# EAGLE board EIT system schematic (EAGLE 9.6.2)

Size 100 x 80 mm. Coordinates in mm from the lower left corner, seen from the top.
Outline: 0,0 100,0 100,80 0,80 0,0
Copper layers (1*16): Top 0.035mm / dielectric 1.5mm / Bottom 0.035mm
Design rules "default": minimum track width 6mil, minimum drill 0.35mm, track to track 6mil, track to pad 6mil, pad to pad 6mil, via to via 6mil, smd to smd 6mil, copper to edge 40mil, drill to drill 6mil, minimum pad ring 10mil, minimum via ring 8mil, stop-mask expansion 4mil, vias tented up to drill 0mil, thermal gap 10mil

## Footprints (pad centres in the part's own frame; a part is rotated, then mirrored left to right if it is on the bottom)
1X02 = drill 1.016 long: 1 -1.27,0; 2 1.27,0
C0805 = smd 1.3 x 1.5: 1 -0.95,0; 2 0.95,0
1X05 = drill 1.016 long: 1 -5.08,0; 2 -2.54,0; 3 0,0; 4 2.54,0; 5 5.08,0
SO14 = smd 0.66 x 2.032: 1 -3.81,-3.073; 2 -2.54,-3.073; 3 -1.27,-3.073; 4 0,-3.073; 5 1.27,-3.073; 6 2.54,-3.073; 7 3.81,-3.073; 8 3.81,3.073; 9 2.54,3.073; 10 1.27,3.073; 11 0,3.073; 12 -1.27,3.073; 13 -2.54,3.073; 14 -3.81,3.073
1X01 = drill 1.016 octagon: 1 0,0
2X16 = drill 1.016 octagon: 1 -19.05,-1.27; 2 -19.05,1.27; 3 -16.51,-1.27; 4 -16.51,1.27; 5 -13.97,-1.27; 6 -13.97,1.27; 7 -11.43,-1.27; 8 -11.43,1.27; 9 -8.89,-1.27; 10 -8.89,1.27; 11 -6.35,-1.27; 12 -6.35,1.27; 13 -3.81,-1.27; 14 -3.81,1.27; 15 -1.27,-1.27; 16 -1.27,1.27; 17 1.27,-1.27; 18 1.27,1.27; 19 3.81,-1.27; 20 3.81,1.27; 21 6.35,-1.27; 22 6.35,1.27; 23 8.89,-1.27; 24 8.89,1.27; 25 11.43,-1.27; 26 11.43,1.27; 27 13.97,-1.27; 28 13.97,1.27; 29 16.51,-1.27; 30 16.51,1.27; 31 19.05,-1.27; 32 19.05,1.27
2X08 = drill 1.016 octagon: 1 -8.89,-1.27; 2 -8.89,1.27; 3 -6.35,-1.27; 4 -6.35,1.27; 5 -3.81,-1.27; 6 -3.81,1.27; 7 -1.27,-1.27; 8 -1.27,1.27; 9 1.27,-1.27; 10 1.27,1.27; 11 3.81,-1.27; 12 3.81,1.27; 13 6.35,-1.27; 14 6.35,1.27; 15 8.89,-1.27; 16 8.89,1.27
1_05X2MM = drill 1.016 pad 1.3 square: 1 -4,0 | drill 1.016 pad 1.3: 2 -2,0; 3 0,0; 4 2,0; 5 4,0
M0805 = smd 1.3 x 1.6: 1 -0.95,0; 2 0.95,0
SOIC127P599X175-8N = smd 1.97 x 0.6: 1 -2.47,1.905; 2 -2.47,0.635; 3 -2.47,-0.635; 4 -2.47,-1.905; 5 2.47,-1.905; 6 2.47,-0.635; 7 2.47,0.635; 8 2.47,1.905
DIP254P762X533-8 = drill 1.118 square: 1 -7.62,7.62 | drill 1.118: 2 -7.62,5.08; 3 -7.62,2.54; 4 -7.62,0; 5 0,0; 6 0,2.54; 7 0,5.08; 8 0,7.62
SOIC127P1030X265-24N = smd 2.06 x 0.6: 1 -4.64,6.985; 2 -4.64,5.715; 3 -4.64,4.445; 4 -4.64,3.175; 5 -4.64,1.905; 6 -4.64,0.635; 7 -4.64,-0.635; 8 -4.64,-1.905; 9 -4.64,-3.175; 10 -4.64,-4.445; 11 -4.64,-5.715; 12 -4.64,-6.985; 13 4.64,-6.985; 14 4.64,-5.715; 15 4.64,-4.445; 16 4.64,-3.175; 17 4.64,-1.905; 18 4.64,-0.635; 19 4.64,0.635; 20 4.64,1.905; 21 4.64,3.175; 22 4.64,4.445; 23 4.64,5.715; 24 4.64,6.985
DIP1016W50P254L742H480Q6 = drill 0.82 square: 1 -5.08,2.54 | drill 0.82: 2 -5.08,0; 3 -5.08,-2.54; 4 5.08,-2.54; 5 5.08,0; 6 5.08,2.54

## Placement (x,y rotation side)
ADC1-2  [1X02]  not placed on the board
C3  1uf  [C0805]  not placed on the board
C4  1uf  [C0805]  not placed on the board
DEMUX3  [1X05]  not placed on the board
DEMUX4  [1X05]  not placed on the board
IC2  7404D  [SO14]  not placed on the board
JP2  [1X01]  74.93,12.7 0 top
JP3  [2X16]  not placed on the board
JP6  [2X08]  not placed on the board
MUX1_2  [1_05X2MM]  not placed on the board
R1  10K  [M0805]  not placed on the board
R2  10k  [M0805]  not placed on the board
R3  10k  [M0805]  not placed on the board
R4  10K  [M0805]  not placed on the board
R5  [M0805]  not placed on the board
R6  10k  [M0805]  not placed on the board
R7  10k  [M0805]  not placed on the board
R8  [M0805]  not placed on the board
R9  [M0805]  not placed on the board
R10  [M0805]  not placed on the board
R11  10K  [M0805]  not placed on the board
R12  10k  [M0805]  not placed on the board
R13  10k  [M0805]  not placed on the board
R14  10K  [M0805]  not placed on the board
R15  [M0805]  not placed on the board
R16  10k  [M0805]  not placed on the board
R17  10k  [M0805]  not placed on the board
R18  10K  [M0805]  not placed on the board
R19  10k  [M0805]  not placed on the board
R20  10k  [M0805]  not placed on the board
R21  [M0805]  not placed on the board
R22  [M0805]  not placed on the board
R23  [M0805]  not placed on the board
R24  [M0805]  not placed on the board
R25  [M0805]  not placed on the board
R26  [M0805]  not placed on the board
R27  [M0805]  not placed on the board
R28  10K  [M0805]  not placed on the board
R29  [M0805]  not placed on the board
R30  10k  [M0805]  not placed on the board
R31  10k  [M0805]  not placed on the board
R32  10K  [M0805]  not placed on the board
R33  10k  [M0805]  not placed on the board
R34  10k  [M0805]  not placed on the board
R35  10K  [M0805]  not placed on the board
R36  [M0805]  not placed on the board
R37  10k  [M0805]  not placed on the board
R38  10k  [M0805]  not placed on the board
R39  10K  [M0805]  not placed on the board
R40  10k  [M0805]  not placed on the board
R41  10k  [M0805]  not placed on the board
R42  10K  [M0805]  not placed on the board
R43  [M0805]  not placed on the board
R44  10k  [M0805]  not placed on the board
R45  10k  [M0805]  not placed on the board
R46  10K  [M0805]  not placed on the board
R47  10k  [M0805]  not placed on the board
R48  10k  [M0805]  not placed on the board
R49  10K  [M0805]  not placed on the board
R50  [M0805]  not placed on the board
R51  10k  [M0805]  not placed on the board
R52  10k  [M0805]  not placed on the board
R53  10K  [M0805]  not placed on the board
R54  10k  [M0805]  not placed on the board
R55  10k  [M0805]  not placed on the board
R56  10K  [M0805]  not placed on the board
R57  [M0805]  not placed on the board
R58  10k  [M0805]  not placed on the board
R59  10k  [M0805]  not placed on the board
R60  10K  [M0805]  not placed on the board
R61  10k  [M0805]  not placed on the board
R62  10k  [M0805]  not placed on the board
R63  10K  [M0805]  not placed on the board
R64  [M0805]  not placed on the board
R65  10k  [M0805]  not placed on the board
R66  10k  [M0805]  not placed on the board
R67  10K  [M0805]  not placed on the board
R68  10k  [M0805]  not placed on the board
R69  10k  [M0805]  not placed on the board
R70  10K  [M0805]  not placed on the board
R71  [M0805]  not placed on the board
R72  10k  [M0805]  not placed on the board
R73  10k  [M0805]  not placed on the board
R74  10K  [M0805]  not placed on the board
R75  10k  [M0805]  not placed on the board
R76  10k  [M0805]  not placed on the board
R77  10K  [M0805]  not placed on the board
R78  [M0805]  not placed on the board
R79  10k  [M0805]  not placed on the board
R80  10k  [M0805]  not placed on the board
R81  10K  [M0805]  not placed on the board
R82  10k  [M0805]  not placed on the board
R83  10k  [M0805]  not placed on the board
R84  10K  [M0805]  not placed on the board
R85  [M0805]  not placed on the board
R86  10k  [M0805]  not placed on the board
R87  10k  [M0805]  not placed on the board
R88  10K  [M0805]  not placed on the board
R89  10k  [M0805]  not placed on the board
R90  10k  [M0805]  not placed on the board
R91  10K  [M0805]  not placed on the board
R92  [M0805]  not placed on the board
R93  10k  [M0805]  not placed on the board
R94  10k  [M0805]  not placed on the board
R95  10K  [M0805]  not placed on the board
R96  10k  [M0805]  not placed on the board
R97  10k  [M0805]  not placed on the board
R98  10K  [M0805]  not placed on the board
R99  [M0805]  not placed on the board
R100  10k  [M0805]  not placed on the board
R101  10k  [M0805]  not placed on the board
R102  10K  [M0805]  not placed on the board
R103  10k  [M0805]  not placed on the board
R104  10k  [M0805]  not placed on the board
R105  10K  [M0805]  not placed on the board
R106  [M0805]  not placed on the board
R107  10k  [M0805]  not placed on the board
R108  10k  [M0805]  not placed on the board
R109  10K  [M0805]  not placed on the board
R110  10k  [M0805]  not placed on the board
R111  10k  [M0805]  not placed on the board
R112  10K  [M0805]  not placed on the board
R113  [M0805]  not placed on the board
R114  10k  [M0805]  not placed on the board
R115  10k  [M0805]  82.55,29.21 0 top
R116  10K  [M0805]  not placed on the board
R117  10k  [M0805]  not placed on the board
R118  10k  [M0805]  not placed on the board
R119  10K  [M0805]  not placed on the board
R120  [M0805]  not placed on the board
R121  10k  [M0805]  not placed on the board
R122  10k  [M0805]  not placed on the board
SUPPLY  [1X02]  not placed on the board
U1  OPA657U  [SOIC127P599X175-8N]  93.98,72.39 0 top
U2  OPA657U  [SOIC127P599X175-8N]  88.9,17.78 0 top
U3  AD781JNZ  [DIP254P762X533-8]  not placed on the board
U4  AD781JNZ  [DIP254P762X533-8]  not placed on the board
U5  OPA657U  [SOIC127P599X175-8N]  45.72,17.78 0 top
U6  OPA657U  [SOIC127P599X175-8N]  44.45,52.07 0 top
U7  OPA657U  [SOIC127P599X175-8N]  not placed on the board
U8  OPA657U  [SOIC127P599X175-8N]  not placed on the board
U9  CD74HCT4067M  [SOIC127P1030X265-24N]  24.13,27.94 0 top
U10  CD74HCT4067M  [SOIC127P1030X265-24N]  not placed on the board
U11  AD781JNZ  [DIP254P762X533-8]  not placed on the board
U12  AD781JNZ  [DIP254P762X533-8]  not placed on the board
U13  AD781JNZ  [DIP254P762X533-8]  not placed on the board
U14  AD781JNZ  [DIP254P762X533-8]  not placed on the board
U15  AD781JNZ  [DIP254P762X533-8]  not placed on the board
U16  AD781JNZ  [DIP254P762X533-8]  not placed on the board
U17  AD781JNZ  [DIP254P762X533-8]  not placed on the board
U18  AD781JNZ  [DIP254P762X533-8]  not placed on the board
U19  AD781JNZ  [DIP254P762X533-8]  not placed on the board
U20  AD781JNZ  [DIP254P762X533-8]  not placed on the board
U21  OPA657U  [SOIC127P599X175-8N]  not placed on the board
U22  AD781JNZ  [DIP254P762X533-8]  not placed on the board
U23  OPA657U  [SOIC127P599X175-8N]  not placed on the board
U24  H11AA4M  [DIP1016W50P254L742H480Q6]  not placed on the board
U25  H11AA4M  [DIP1016W50P254L742H480Q6]  not placed on the board
U26  CD74HCT4067M  [SOIC127P1030X265-24N]  not placed on the board
U27  CD74HCT4067M  [SOIC127P1030X265-24N]  not placed on the board
U28  OPA657U  [SOIC127P599X175-8N]  not placed on the board
U29  OPA657U  [SOIC127P599X175-8N]  not placed on the board
U30  OPA657U  [SOIC127P599X175-8N]  not placed on the board
U31  OPA657U  [SOIC127P599X175-8N]  not placed on the board
U32  OPA657U  [SOIC127P599X175-8N]  not placed on the board
U33  OPA657U  [SOIC127P599X175-8N]  not placed on the board
U34  OPA657U  [SOIC127P599X175-8N]  not placed on the board
U35  OPA657U  [SOIC127P599X175-8N]  60.96,12.7 0 top
U36  OPA657U  [SOIC127P599X175-8N]  17.78,67.31 0 top
U37  OPA657U  [SOIC127P599X175-8N]  44.45,69.85 0 top
U38  OPA657U  [SOIC127P599X175-8N]  not placed on the board
U39  OPA657U  [SOIC127P599X175-8N]  not placed on the board
U40  AD781JNZ  [DIP254P762X533-8]  not placed on the board
U41  AD781JNZ  [DIP254P762X533-8]  not placed on the board
U42  AD781JNZ  [DIP254P762X533-8]  not placed on the board
U43  AD781JNZ  [DIP254P762X533-8]  not placed on the board
U44  AD781JNZ  [DIP254P762X533-8]  not placed on the board
U45  AD781JNZ  [DIP254P762X533-8]  not placed on the board
U46  AD781JNZ  [DIP254P762X533-8]  not placed on the board
U47  AD781JNZ  [DIP254P762X533-8]  not placed on the board
U48  AD781JNZ  [DIP254P762X533-8]  not placed on the board
U49  AD781JNZ  [DIP254P762X533-8]  not placed on the board
U50  AD781JNZ  [DIP254P762X533-8]  not placed on the board
U51  AD781JNZ  [DIP254P762X533-8]  not placed on the board
U52  AD781JNZ  [DIP254P762X533-8]  not placed on the board
U53  AD781JNZ  [DIP254P762X533-8]  not placed on the board
U54  AD781JNZ  [DIP254P762X533-8]  not placed on the board
U55  AD781JNZ  [DIP254P762X533-8]  not placed on the board
U56  AD781JNZ  [DIP254P762X533-8]  not placed on the board
U57  AD781JNZ  [DIP254P762X533-8]  not placed on the board
U58  AD781JNZ  [DIP254P762X533-8]  not placed on the board
U59  OPA657U  [SOIC127P599X175-8N]  not placed on the board
U60  OPA657U  [SOIC127P599X175-8N]  not placed on the board
U61  OPA657U  [SOIC127P599X175-8N]  not placed on the board
U62  OPA657U  [SOIC127P599X175-8N]  not placed on the board
U63  OPA657U  [SOIC127P599X175-8N]  not placed on the board
U64  OPA657U  [SOIC127P599X175-8N]  not placed on the board
U65  OPA657U  [SOIC127P599X175-8N]  not placed on the board
U66  OPA657U  [SOIC127P599X175-8N]  not placed on the board
U67  OPA657U  [SOIC127P599X175-8N]  not placed on the board
U68  OPA657U  [SOIC127P599X175-8N]  91.44,60.96 0 top
U69  OPA657U  [SOIC127P599X175-8N]  83.82,72.39 0 top
U70  OPA657U  [SOIC127P599X175-8N]  57.15,71.12 0 top
U71  OPA657U  [SOIC127P599X175-8N]  not placed on the board
U72  OPA657U  [SOIC127P599X175-8N]  not placed on the board
U73  OPA657U  [SOIC127P599X175-8N]  not placed on the board
U74  OPA657U  [SOIC127P599X175-8N]  not placed on the board
U75  OPA657U  [SOIC127P599X175-8N]  not placed on the board
U76  OPA657U  [SOIC127P599X175-8N]  not placed on the board
U77  OPA657U  [SOIC127P599X175-8N]  not placed on the board
U78  OPA657U  [SOIC127P599X175-8N]  not placed on the board
U79  OPA657U  [SOIC127P599X175-8N]  not placed on the board
U80  OPA657U  [SOIC127P599X175-8N]  not placed on the board
U81  OPA657U  [SOIC127P599X175-8N]  not placed on the board
U82  OPA657U  [SOIC127P599X175-8N]  not placed on the board
U83  OPA657U  [SOIC127P599X175-8N]  71.12,71.12 0 top
U84  OPA657U  [SOIC127P599X175-8N]  31.75,68.58 0 top
U85  OPA657U  [SOIC127P599X175-8N]  81.28,48.26 0 top
U86  OPA657U  [SOIC127P599X175-8N]  not placed on the board
U87  OPA657U  [SOIC127P599X175-8N]  not placed on the board
U88  OPA657U  [SOIC127P599X175-8N]  not placed on the board

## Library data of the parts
ADC1-2 DEMUX3 DEMUX4 JP2 JP3 JP6 MUX1_2 SUPPLY = pinhead
C3 C4 = rcl; SPICEPREFIX: C
IC2 = 74xx-eu
R1-R122 = rcl; SPICEPREFIX: R
U1 U2 U5-U8 U21 U23 U28-U39 U59-U88 = OPA657U; DESCRIPTION: 1.6GHz, Low Noise, FET-Input Operational Amplifier 8-SOIC -40 to 85; DIGI-KEY_PART_NUMBER: OPA657UB-ND; MF: Texas Instruments; MP: OPA657U; PACKAGE: SOIC-8 Texas Instruments; PURCHASE-URL: https://pricing.snapeda.com/search/part/OPA657U/?ref=eda
U3 U4 U11-U20 U22 U40-U58 = AD781JNZ; AVAILABILITY: Good; DESCRIPTION: Sample and Hold Amplifier 1 Circuit 8-PDIP; MF: Analog Devices; MP: AD781JNZ; PACKAGE: PDIP-8 Analog Devices; PRICE: None; PURCHASE-URL: https://pricing.snapeda.com/search/part/AD781JNZ/?ref=eda
U9 U10 U26 U27 = CD74HCT4067M; AVAILABILITY: Good; DESCRIPTION: 5-V, 16:1, 1-channel analog multiplexer with TTL inputs 24-SOIC -55 to 125; MF: Texas Instruments; MP: CD74HCT4067M; PACKAGE: SOIC-24 Texas Instruments; PRICE: None; PURCHASE-URL: https://pricing.snapeda.com/search/part/CD74HCT4067M/?ref=eda
U24 U25 = H11AA4M; AVAILABILITY: Good; DESCRIPTION: AC-IN 1-CH Transistor With Base DC-OUT 6-Pin PDIP Bag; MF: ON Semiconductor; MP: H11AA4M; PACKAGE: PDIP-6 ON Semiconductor; PRICE: None; PURCHASE-URL: https://pricing.snapeda.com/search/part/H11AA4M/?ref=eda

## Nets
0: C3.1 C4.1 R7.1 R17.1 R22.2 R23.2 R31.1 R38.1 R45.1 R52.1 R59.1 R66.1 R73.1 R80.1 R87.1 R94.1 R101.1 R108.1 R115.1 R122.1 U3.3 U4.3 U9.12 U10.12 U11.3 U12.3 U13.3 U14.3 U15.3 U16.3 U17.3 U18.3 U19.3 U20.3 U22.3 U24.2 U25.2 U26.12 U27.12 U40.3 U41.3 U42.3 U43.3 U44.3 U45.3 U46.3 U47.3 U48.3 U49.3 U50.3 U51.3 U52.3 U53.3 U54.3 U55.3 U56.3 U57.3 U58.3
+5V: U27.24
+12V: C4.2 SUPPLY.1 U13.1 U14.1 U17.1 U20.1 U40.1 U41.1 U42.1 U44.1 U45.1 U46.1 U47.1 U48.1 U53.1 U54.1 U55.1 U56.1
-5V: U21.4
-12V: C3.2 SUPPLY.2 U13.5 U14.5 U17.5 U20.5 U40.5 U41.5 U42.5 U44.5 U45.5 U46.5 U47.5 U48.5 U49.1 U53.5 U54.5 U55.5 U56.5
D3E: DEMUX3.1
D3S0: DEMUX3.2 U9.10
D3S1: DEMUX3.3 U9.11
D3S2: DEMUX3.4 U9.14
D3S3: DEMUX3.5 U9.13
D4E: DEMUX4.1
D4S0: DEMUX4.2
D4S1: DEMUX4.3
D4S2: DEMUX4.4
D4S3: DEMUX4.5
E: MUX1_2.1 U26.15
GND: IC2.7
I0: JP3.2 U48.8
I1: JP3.4 U10.8 U45.8
I2: JP3.6 U10.7 U53.8
I3: JP3.8 U10.6 U44.8
I4: JP3.10 U10.5 U46.8
I5: JP3.12 U10.4 U12.8
I6: JP3.14 U4.8 U10.3
I7: JP3.16 U3.8 U10.2
I8: JP3.18 U10.23 U22.8
I9: JP3.20 U10.22 U18.8
I10: JP3.22 U10.21 U57.8
I11: JP3.24 U10.20 U50.8
I12: JP3.26 U10.19 U51.8
I13: JP3.28 U10.18 U43.8
I14: JP3.30 U10.17 U58.8
I15: JP3.32 U10.16 U52.8
IO: U10.9
M1I0: U26.9 U48.2
M1I1: U26.8 U45.2
M1I2: U26.7 U53.2
M1I3: U26.6 U44.2
M1I4: U26.5 U46.2
M1I5: U12.2 U26.4
M1I6: U4.2 U26.3
M1I7: U3.2 U26.2
M1I8: U22.2 U26.23
M1I9: U18.2 U26.22
M1I10: U26.21 U57.2
M1I11: U26.20 U50.2
M1I12: U26.19 U51.2
M1I13: U26.18 U43.2
M1I14: U26.17 U58.2
M1I15: U26.16 U52.2
M2I0: U11.2 U27.9
M2I1: U15.2 U27.8
M2I2: U14.2 U27.7
M2I3: U13.2 U27.6
M2I4: U27.5 U54.2
M2I5: U27.4 U40.2
M2I6: U27.3 U47.2
M2I7: U27.2 U55.2
M2I8: U19.2 U27.23
M2I9: U16.2 U27.22
M2I10: U17.2 U27.21
M2I11: U20.2 U27.20
M2I12: U27.19 U56.2
M2I13: U27.18 U49.2
M2I14: U27.17 U42.2
M2I15: U27.16 U41.2
N$1: U9.24
N$3: U1.4
N$4: U1.7
N$5: U2.4
N$6: U2.7
N$7: U5.4
N$8: U5.7
N$9: U23.4
N$10: U23.7
N$11: U25.4 U27.1
N$12: ADC1-2.2 U10.1
N$14: IC2.1 JP2.1
N$15: U41.7
N$16: U52.1
N$17: JP3.1 U11.8
N$18: R2.1 R3.2 U2.2
N$19: JP3.3 U15.8
N$20: R1.1 R2.2 U1.2
N$21: JP3.5 U14.8
N$22: R3.1 R5.2 U2.6
N$23: JP3.7 U13.8
N$24: R5.1 R7.2 U5.3
N$25: U40.7
N$26: JP3.17 U19.8
N$27: JP3.19 U16.8
N$28: R1.2 R4.2 U1.6
N$29: R4.1 R6.2 U5.2
N$30: U4.7
N$31: U49.5
N$32: U4.1
N$33: JP3.21 U17.8
N$34: R6.1 U5.6 U9.22
N$35: JP3.23 U20.8
N$36: JP3.25 U56.8
N$37: JP3.27 U49.8
N$39: U4.5
N$40: U3.1
N$41: U3.7
N$43: U53.7
N$45: U44.7
N$47: U46.7
N$49: U12.1
N$50: U12.7
N$51: U12.5
N$54: U3.5
N$55: U11.1
N$56: U11.7
N$57: U42.7
N$58: U11.5
N$59: U15.1
N$60: U15.7
N$61: U52.7
N$62: U15.5
N$63: U14.7
N$64: U52.5
N$65: U49.7
N$66: U56.7
N$67: U54.7
N$68: U13.7
N$69: U58.1
N$70: U55.7
N$71: U47.7
N$72: U20.7
N$73: JP3.9 U54.8
N$74: JP3.11 U40.8
N$75: JP3.13 U47.8
N$76: JP3.15 U55.8
N$77: U58.7
N$78: U17.7
N$79: U6.4
N$80: U16.1
N$81: U16.7
N$82: U58.5
N$83: U16.5
N$84: U19.1
N$85: U19.7
N$86: U43.1
N$87: U19.5
N$88: JP3.29 U42.8
N$89: JP3.31 U41.8
N$90: U43.7
N$91: U6.7
N$92: U43.5
N$93: U51.1
N$94: U51.7
N$95: U7.4
N$96: U51.5
N$97: U50.1
N$98: U50.7
N$99: U7.7
N$100: U50.5
N$101: U57.1
N$102: U57.7
N$103: U8.4
N$104: U57.5
N$105: U18.1
N$106: U18.7
N$107: U8.7
N$108: U18.5
N$109: U22.1
N$110: U22.7
N$111: R37.1 U9.7 U33.6
N$112: U22.5
N$121: R8.2 R10.1 U21.3
N$122: R21.2 R22.1 U21.2
N$123: R9.2 R21.1 U21.6
N$124: R8.1 R9.1 U24.1
N$125: R23.1 R26.2 U23.3
N$126: R24.1 R27.2 U23.2
N$127: R25.2 R27.1 U23.6
N$128: R25.1 R26.1 U25.1
N$129: R24.2
N$130: U25.5
N$131: U24.4 U26.1
N$132: U80.4
N$133: U27.10
N$134: U27.11
N$135: U27.15
N$136: U27.14
N$137: U27.13
N$138: R93.1 U9.8 U76.6
N$139: R12.1 R13.2 U7.2
N$140: R11.1 R12.2 U6.2
N$141: R13.1 R15.2 U7.6
N$142: R15.1 R17.2 U8.3
N$143: R11.2 R14.2 U6.6
N$144: R14.1 R16.2 U8.2
N$145: R16.1 U8.6 U9.18
N$146: U28.4
N$147: U28.7
N$148: U29.4
N$149: U29.7
N$150: U30.4
N$151: U30.7
N$152: R86.1 U9.9 U73.6
N$153: U10.24
N$154: R19.1 R20.2 U29.2
N$155: R18.1 R19.2 U28.2
N$156: R20.1 R29.2 U29.6
N$157: R29.1 R31.2 U30.3
N$158: R18.2 R28.2 U28.6
N$159: R28.1 R30.2 U30.2
N$160: R30.1 U9.3 U30.6
N$161: U31.4
N$162: U31.7
N$163: U32.4
N$164: U32.7
N$165: U33.4
N$166: U33.7
N$167: U10.10
N$168: U10.11
N$169: R33.1 R34.2 U32.2
N$170: R32.1 R33.2 U31.2
N$171: R34.1 R36.2 U32.6
N$172: R36.1 R38.2 U33.3
N$173: R32.2 R35.2 U31.6
N$174: R35.1 R37.2 U33.2
N$175: U10.13
N$176: U34.4
N$177: U34.7
N$178: U35.4
N$179: U35.7
N$180: U36.4
N$181: U36.7
N$182: U10.14
N$184: R40.1 R41.2 U35.2
N$185: R39.1 R40.2 U34.2
N$186: R41.1 R43.2 U35.6
N$187: R43.1 R45.2 U36.3
N$188: R39.2 R42.2 U34.6
N$189: R42.1 R44.2 U36.2
N$190: R44.1 U9.21 U36.6
N$191: U37.4
N$192: U37.7
N$193: U38.4
N$194: U38.7
N$195: U39.4
N$196: U39.7
N$199: R47.1 R48.2 U38.2
N$200: R46.1 R47.2 U37.2
N$201: R48.1 R50.2 U38.6
N$202: R50.1 R52.2 U39.3
N$203: R46.2 R49.2 U37.6
N$204: R49.1 R51.2 U39.2
N$205: R51.1 U9.20 U39.6
N$206: U59.4
N$207: U59.7
N$208: U60.4
N$209: U60.7
N$210: U61.4
N$211: U61.7
N$214: R54.1 R55.2 U60.2
N$215: R53.1 R54.2 U59.2
N$216: R55.1 R57.2 U60.6
N$217: R57.1 R59.2 U61.3
N$218: R53.2 R56.2 U59.6
N$219: R56.1 R58.2 U61.2
N$220: R58.1 U9.16 U61.6
N$221: U62.4
N$222: U62.7
N$223: U63.4
N$224: U63.7
N$225: U64.4
N$226: U64.7
N$229: R61.1 R62.2 U63.2
N$230: R60.1 R61.2 U62.2
N$231: R62.1 R64.2 U63.6
N$232: R64.1 R66.2 U64.3
N$233: R60.2 R63.2 U62.6
N$234: R63.1 R65.2 U64.2
N$235: R65.1 U9.17 U64.6
N$236: U65.4
N$237: U65.7
N$238: U66.4
N$239: U66.7
N$240: U67.4
N$241: U67.7
N$244: R68.1 R69.2 U66.2
N$245: R67.1 R68.2 U65.2
N$246: R69.1 R71.2 U66.6
N$247: R71.1 R73.2 U67.3
N$248: R67.2 R70.2 U65.6
N$249: R70.1 R72.2 U67.2
N$250: R72.1 U9.4 U67.6
N$251: U68.4
N$252: U68.7
N$253: U69.4
N$254: U69.7
N$255: U70.4
N$256: U70.7
N$259: R75.1 R76.2 U69.2
N$260: R74.1 R75.2 U68.2
N$261: R76.1 R78.2 U69.6
N$262: R78.1 R80.2 U70.3
N$263: R74.2 R77.2 U68.6
N$264: R77.1 R79.2 U70.2
N$265: R79.1 U9.5 U70.6
N$266: U71.4
N$267: U71.7
N$268: U72.4
N$269: U72.7
N$270: U73.4
N$271: U73.7
N$274: R82.1 R83.2 U72.2
N$275: R81.1 R82.2 U71.2
N$276: R83.1 R85.2 U72.6
N$277: R85.1 R87.2 U73.3
N$278: R81.2 R84.2 U71.6
N$279: R84.1 R86.2 U73.2
N$281: U74.4
N$282: U74.7
N$283: U75.4
N$284: U75.7
N$285: U76.4
N$286: U76.7
N$289: R89.1 R90.2 U75.2
N$290: R88.1 R89.2 U74.2
N$291: R90.1 R92.2 U75.6
N$292: R92.1 R94.2 U76.3
N$293: R88.2 R91.2 U74.6
N$294: R91.1 R93.2 U76.2
N$296: U77.4
N$297: U77.7
N$298: U21.7
N$299: U78.4
N$300: U78.7
N$301: U79.4
N$302: U79.7
N$305: R96.1 R97.2 U78.2
N$306: R95.1 R96.2 U77.2
N$307: R97.1 R99.2 U78.6
N$308: R99.1 R101.2 U79.3
N$309: R95.2 R98.2 U77.6
N$310: R98.1 R100.2 U79.2
N$311: R100.1 U9.23 U79.6
N$312: U80.7
N$313: U81.4
N$314: U81.7
N$315: U82.4
N$316: U82.7
N$319: R103.1 R104.2 U81.2
N$320: R102.1 R103.2 U80.2
N$321: R104.1 R106.2 U81.6
N$322: R106.1 R108.2 U82.3
N$323: R102.2 R105.2 U80.6
N$324: R105.1 R107.2 U82.2
N$325: R107.1 U9.19 U82.6
N$326: U83.4
N$327: U83.7
N$328: U84.4
N$329: U84.7
N$330: U85.4
N$331: U85.7
N$334: R110.1 R111.2 U84.2
N$335: R109.1 R110.2 U83.2
N$336: R111.1 R113.2 U84.6
N$337: R113.1 R115.2 U85.3
N$338: R109.2 R112.2 U83.6
N$339: R112.1 R114.2 U85.2
N$340: R114.1 U9.2 U85.6
N$341: U86.4
N$342: U86.7
N$343: U87.4
N$344: U87.7
N$345: U88.4
N$346: U88.7
N$349: R117.1 R118.2 U87.2
N$350: R116.1 R117.2 U86.2
N$351: R118.1 R120.2 U87.6
N$352: R120.1 R122.2 U88.3
N$353: R116.2 R119.2 U86.6
N$354: R119.1 R121.2 U88.2
N$355: R121.1 U9.6 U88.6
N$361: ADC1-2.1 U9.1
N$367: U9.15
S0: MUX1_2.2 U26.10
S1: MUX1_2.3 U26.11
S2: MUX1_2.4 U26.14
S3: MUX1_2.5 U26.13
STATUS: IC2.2 U45.7 U48.7
V1: JP6.1 U72.3 U77.3
V2: JP6.2 U78.3 U80.3
V3: JP6.3 U81.3 U83.3
V4: JP6.4 U84.3 U86.3
V5: JP6.5 U1.3 U87.3
V6: JP6.6 U2.3 U6.3
V7: JP6.7 U7.3 U28.3
V8: JP6.8 U29.3 U31.3
V9: JP6.9 U32.3 U34.3
V10: JP6.10 U35.3 U62.3
V11: JP6.11 U63.3 U65.3
V12: JP6.12 U66.3 U74.3
V13: JP6.13 U37.3 U75.3
V14: JP6.14 U38.3 U59.3
V15: JP6.15 U60.3 U68.3
V16: JP6.16 U69.3 U71.3
VCC: IC2.14 U26.24
VSOURCE: R10.2 U24.5

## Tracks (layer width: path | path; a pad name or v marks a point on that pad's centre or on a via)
0  (57 unrouted)
+12V  (17 unrouted)
-12V  (18 unrouted)
D3S0  (1 unrouted)
D3S1  (1 unrouted)
D3S2  (1 unrouted)
D3S3  (1 unrouted)
E  (1 unrouted)
I0  (1 unrouted)
I1  (2 unrouted)
I2  (2 unrouted)
I3  (2 unrouted)
I4  (2 unrouted)
I5  (2 unrouted)
I6  (2 unrouted)
I7  (2 unrouted)
I8  (2 unrouted)
I9  (2 unrouted)
I10  (2 unrouted)
I11  (2 unrouted)
I12  (2 unrouted)
I13  (2 unrouted)
I14  (2 unrouted)
I15  (2 unrouted)
M1I0  (1 unrouted)
M1I1  (1 unrouted)
M1I2  (1 unrouted)
M1I3  (1 unrouted)
M1I4  (1 unrouted)
M1I5  (1 unrouted)
M1I6  (1 unrouted)
M1I7  (1 unrouted)
M1I8  (1 unrouted)
M1I9  (1 unrouted)
M1I10  (1 unrouted)
M1I11  (1 unrouted)
M1I12  (1 unrouted)
M1I13  (1 unrouted)
M1I14  (1 unrouted)
M1I15  (1 unrouted)
M2I0  (1 unrouted)
M2I1  (1 unrouted)
M2I2  (1 unrouted)
M2I3  (1 unrouted)
M2I4  (1 unrouted)
M2I5  (1 unrouted)
M2I6  (1 unrouted)
M2I7  (1 unrouted)
M2I8  (1 unrouted)
M2I9  (1 unrouted)
M2I10  (1 unrouted)
M2I11  (1 unrouted)
M2I12  (1 unrouted)
M2I13  (1 unrouted)
M2I14  (1 unrouted)
M2I15  (1 unrouted)
N$11  (1 unrouted)
N$12  (1 unrouted)
N$14  (1 unrouted)
N$17  (1 unrouted)
N$18  (2 unrouted)
N$19  (1 unrouted)
N$20  (2 unrouted)
N$21  (1 unrouted)
N$22  (2 unrouted)
N$23  (1 unrouted)
N$24  (2 unrouted)
N$26  (1 unrouted)
N$27  (1 unrouted)
N$28  (2 unrouted)
N$29  (2 unrouted)
N$33  (1 unrouted)
N$34  (2 unrouted)
N$35  (1 unrouted)
N$36  (1 unrouted)
N$37  (1 unrouted)
N$73  (1 unrouted)
N$74  (1 unrouted)
N$75  (1 unrouted)
N$76  (1 unrouted)
N$88  (1 unrouted)
N$89  (1 unrouted)
N$111  (2 unrouted)
N$121  (2 unrouted)
N$122  (2 unrouted)
N$123  (2 unrouted)
N$124  (2 unrouted)
N$125  (2 unrouted)
N$126  (2 unrouted)
N$127  (2 unrouted)
N$128  (2 unrouted)
N$131  (1 unrouted)
N$138  (2 unrouted)
N$139  (2 unrouted)
N$140  (2 unrouted)
N$141  (2 unrouted)
N$142  (2 unrouted)
N$143  (2 unrouted)
N$144  (2 unrouted)
N$145  (2 unrouted)
N$152  (2 unrouted)
N$154  (2 unrouted)
N$155  (2 unrouted)
N$156  (2 unrouted)
N$157  (2 unrouted)
N$158  (2 unrouted)
N$159  (2 unrouted)
N$160  (2 unrouted)
N$169  (2 unrouted)
N$170  (2 unrouted)
N$171  (2 unrouted)
N$172  (2 unrouted)
N$173  (2 unrouted)
N$174  (2 unrouted)
N$184  (2 unrouted)
N$185  (2 unrouted)
N$186  (2 unrouted)
N$187  (2 unrouted)
N$188  (2 unrouted)
N$189  (2 unrouted)
N$190  (2 unrouted)
N$199  (2 unrouted)
N$200  (2 unrouted)
N$201  (2 unrouted)
N$202  (2 unrouted)
N$203  (2 unrouted)
N$204  (2 unrouted)
N$205  (2 unrouted)
N$214  (2 unrouted)
N$215  (2 unrouted)
N$216  (2 unrouted)
N$217  (2 unrouted)
N$218  (2 unrouted)
N$219  (2 unrouted)
N$220  (2 unrouted)
N$229  (2 unrouted)
N$230  (2 unrouted)
N$231  (2 unrouted)
N$232  (2 unrouted)
N$233  (2 unrouted)
N$234  (2 unrouted)
N$235  (2 unrouted)
N$244  (2 unrouted)
N$245  (2 unrouted)
N$246  (2 unrouted)
N$247  (2 unrouted)
N$248  (2 unrouted)
N$249  (2 unrouted)
N$250  (2 unrouted)
N$259  (2 unrouted)
N$260  (2 unrouted)
N$261  (2 unrouted)
N$262  (2 unrouted)
N$263  (2 unrouted)
N$264  (2 unrouted)
N$265  (2 unrouted)
N$274  (2 unrouted)
N$275  (2 unrouted)
N$276  (2 unrouted)
N$277  (2 unrouted)
N$278  (2 unrouted)
N$279  (2 unrouted)
N$289  (2 unrouted)
N$290  (2 unrouted)
N$291  (2 unrouted)
N$292  (2 unrouted)
N$293  (2 unrouted)
N$294  (2 unrouted)
N$305  (2 unrouted)
N$306  (2 unrouted)
N$307  (2 unrouted)
N$308  (2 unrouted)
N$309  (2 unrouted)
N$310  (2 unrouted)
N$311  (2 unrouted)
N$319  (2 unrouted)
N$320  (2 unrouted)
N$321  (2 unrouted)
N$322  (2 unrouted)
N$323  (2 unrouted)
N$324  (2 unrouted)
N$325  (2 unrouted)
N$334  (2 unrouted)
N$335  (2 unrouted)
N$336  (2 unrouted)
N$337  (2 unrouted)
N$338  (2 unrouted)
N$339  (2 unrouted)
N$340  (2 unrouted)
N$349  (2 unrouted)
N$350  (2 unrouted)
N$351  (2 unrouted)
N$352  (2 unrouted)
N$353  (2 unrouted)
N$354  (2 unrouted)
N$355  (2 unrouted)
N$361  (1 unrouted)
S0  (1 unrouted)
S1  (1 unrouted)
S2  (1 unrouted)
S3  (1 unrouted)
STATUS  (2 unrouted)
V1  (2 unrouted)
V2  (2 unrouted)
V3  (2 unrouted)
V4  (2 unrouted)
V5  (2 unrouted)
V6  (2 unrouted)
V7  (2 unrouted)
V8  (2 unrouted)
V9  (2 unrouted)
V10  (2 unrouted)
V11  (2 unrouted)
V12  (2 unrouted)
V13  (2 unrouted)
V14  (2 unrouted)
V15  (2 unrouted)
V16  (2 unrouted)
VCC  (1 unrouted)
VSOURCE  (1 unrouted)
